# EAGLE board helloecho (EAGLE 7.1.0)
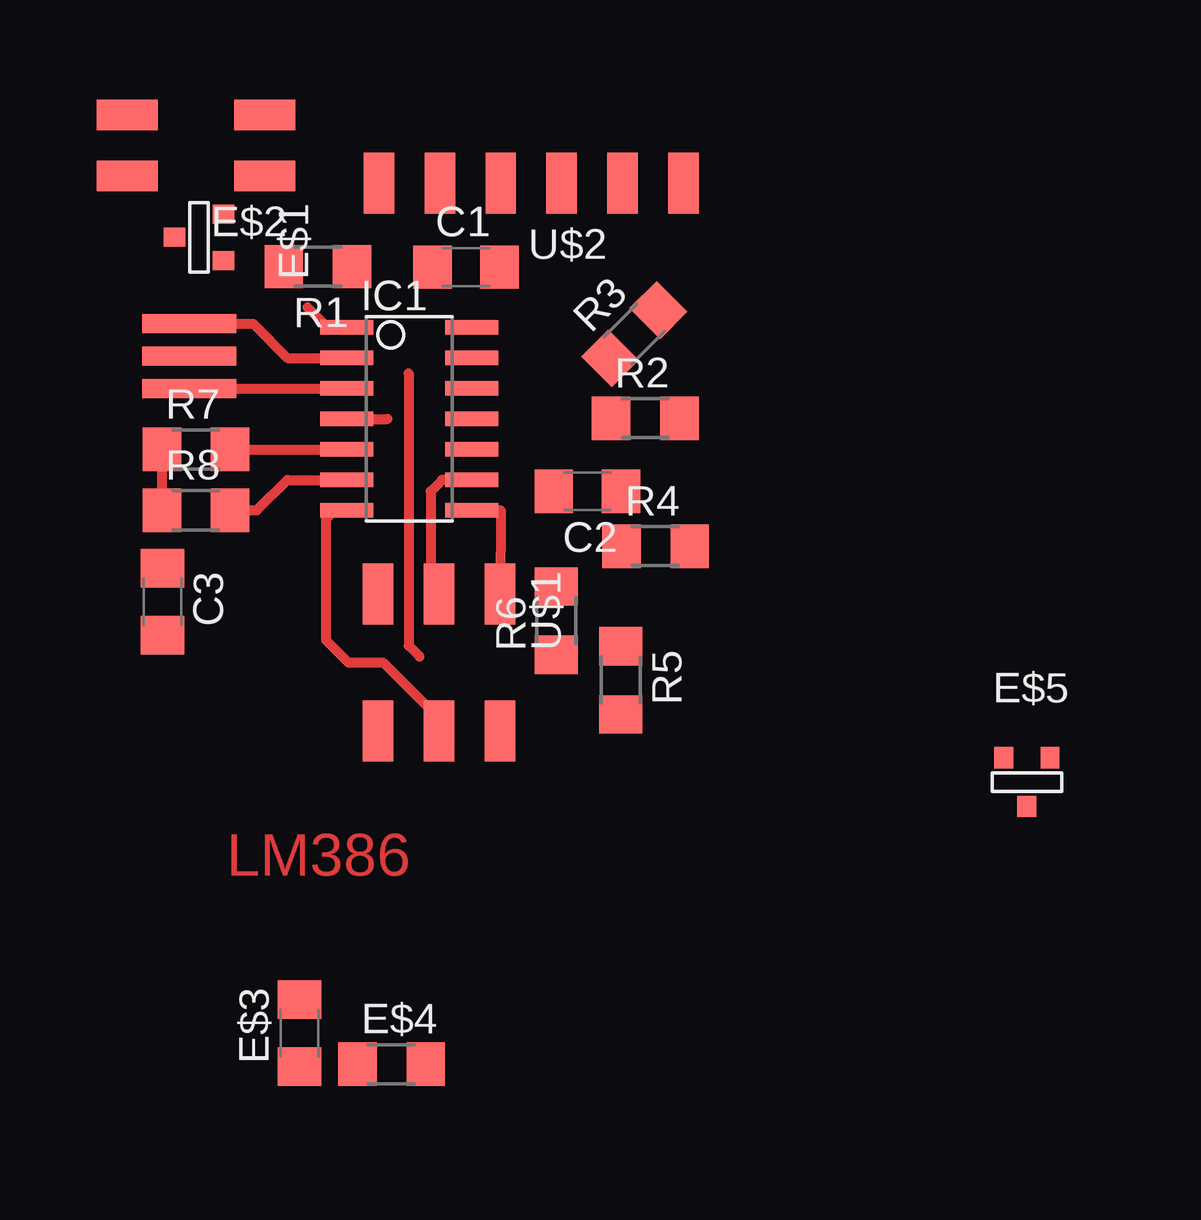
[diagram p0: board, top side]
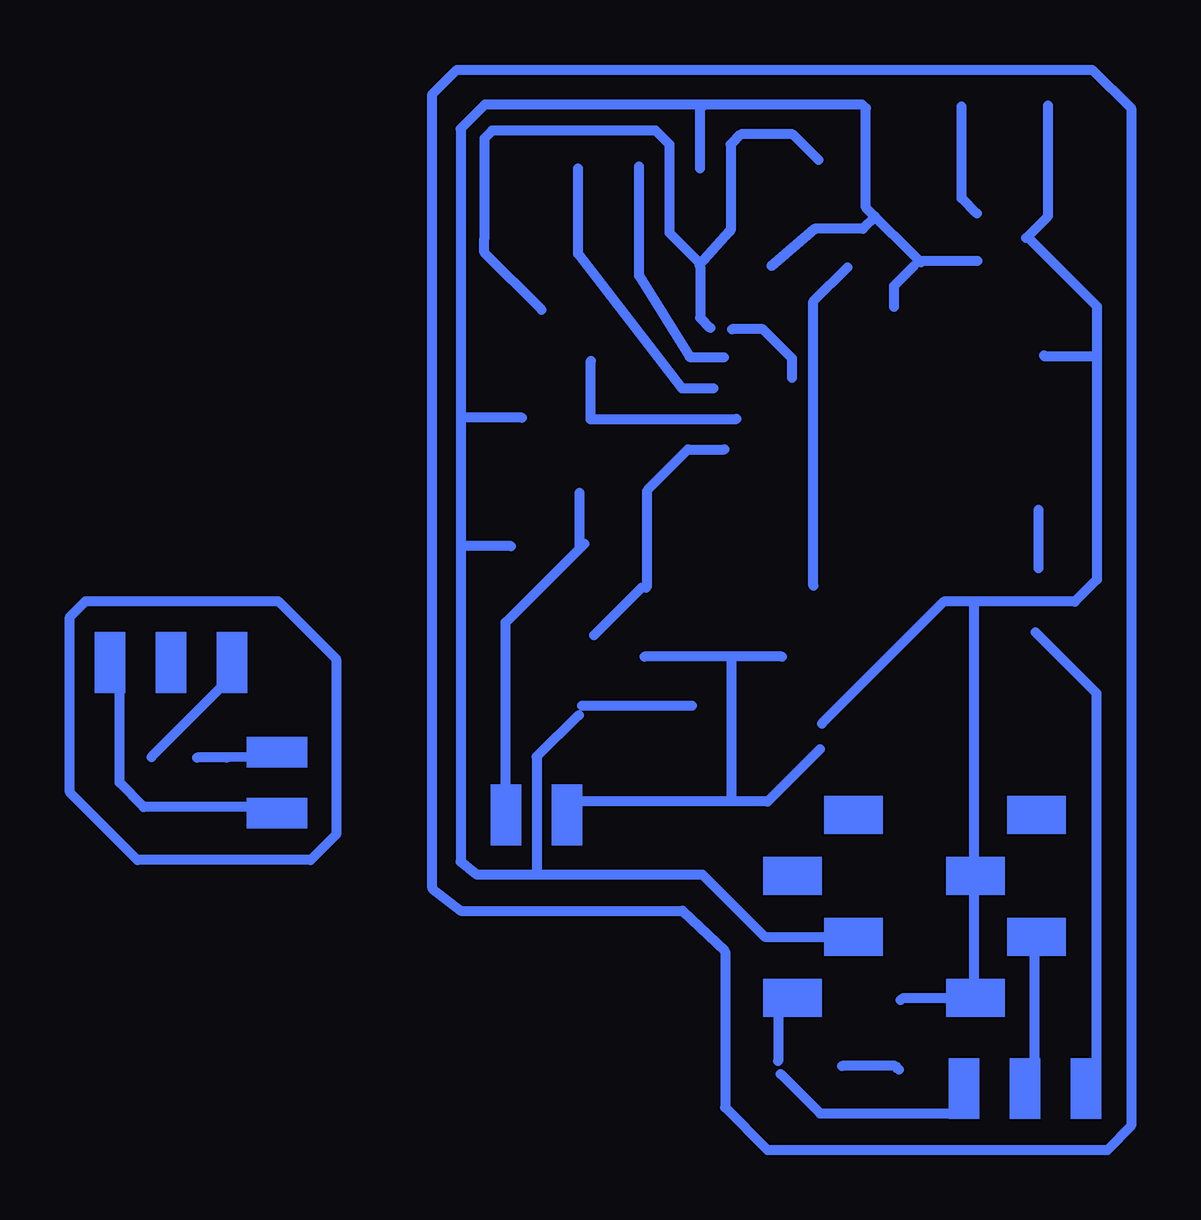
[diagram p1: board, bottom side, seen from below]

No outline drawn. Coordinates in mm, seen from the top.
Copper layers (1*16): Top 0.035mm / dielectric 1.5mm / Bottom 0.035mm
Design rules "default": minimum track width 10mil, minimum drill 24mil, track to track 8mil, track to pad 8mil, pad to pad 8mil, via to via 8mil, smd to smd 8mil, copper to edge 40mil, drill to drill 8mil, minimum pad ring 10mil, minimum via ring 8mil, stop-mask expansion 4mil, vias tented up to drill 0mil, thermal gap 10mil

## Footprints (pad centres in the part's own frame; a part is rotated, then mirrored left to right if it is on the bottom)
EFOBM = smd 0.8 x 3.9: 1 -1.35,0; 2 0,0; 3 1.35,0
C1206 = smd 1.6 x 1.8: 1 -1.4,0; 2 1.4,0
SOT-23 = smd 0.787 x 0.889: 1 0.025,-1.016; 2 -0.94,1.016; 3 0.991,1.016
2X02SMD = smd 2.54 x 1.27: 1 -2.857,1.27; 2 2.857,1.27; 3 -2.857,-1.27; 4 2.857,-1.27
R1206 = smd 1.6 x 1.803: 1 -1.422,0; 2 1.422,0
SOIC14 = smd 0.61 x 2.21: 1 -3.81,-2.603; 2 -2.54,-2.603; 3 -1.27,-2.603; 4 0,-2.603; 5 1.27,-2.603; 6 2.54,-2.603; 7 3.81,-2.603; 8 3.81,2.603; 9 2.54,2.603; 10 1.27,2.603; 11 0,2.603; 12 -1.27,2.603; 13 -2.54,2.603; 14 -3.81,2.603
2X03SMD = smd 2.54 x 1.27: 1 -2.857,2.54; 2 2.857,2.54; 3 -2.857,0; 4 2.857,0; 5 -2.857,-2.54; 6 2.857,-2.54
1X06SMD = smd 2.54 x 1.27: 1 0,6.35; 2 0,3.81; 3 0,1.27; 4 0,-1.27; 5 0,-3.81; 6 0,-6.35

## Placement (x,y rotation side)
20MHZ  RESONATOR  [EFOBM]  18.77,35.64 270 top
C1  1uF  [C1206]  30.3,39.34 0 top
C2  0.1uF  [C1206]  35.36,30 180 top
C3  2.2uF  [C1206]  17.65,25.4 270 top
E$1  REG  [SOT-23]  19.18,40.61 270 top
E$2  [2X02SMD]  19.05,44.42 180 top
E$3  0.1uF  [C1206]  23.37,7.42 90 top
E$4  5  [R1206]  27.2,6.12 0 top
E$5  REG  [SOT-23]  53.64,17.88 0 top
IC1  ATTINY44-SSU  [SOIC14]  27.94,33.02 270 top
R1  10k  [R1206]  24.13,39.37 180 top
R2  10k  [R1206]  37.77,33.05 0 top
R3  10k  [R1206]  37.31,36.55 45 top
R4  10k  [R1206]  38.2,27.71 0 top
R5  10k  [R1206]  36.75,22.12 270 top
R6  10k  [R1206]  34.06,24.61 90 top
R7  1k  [R1206]  19.05,31.75 0 top
R8  255k  [R1206]  19.05,29.21 0 top
U$1  AVRISPSMD  [2X03SMD]  29.18,22.86 270 top
U$2  FTDI-SMD-HEADER  [1X06SMD]  33.02,42.85 90 top

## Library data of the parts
20MHZ C1-C3 E$1-E$5 IC1 R1-R8 U$1 U$2 = fab

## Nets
CTS: U$2.2
MISO: IC1.8 U$1.1
MOSI: IC1.7 U$1.4
N$1: 20MHZ.1 IC1.2
N$2: 20MHZ.3 IC1.3
N$5: R7.1 R8.1
OUT_HI: IC1.5 R7.2
OUT_LO: IC1.6 R8.2
RST: IC1.4
RTS: U$2.6
S$7: IC1.1
S$24: U$1.2
S$36: IC1.14
S$39: U$1.5
SCK: IC1.9 U$1.3

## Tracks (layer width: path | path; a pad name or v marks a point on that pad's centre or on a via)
MISO
  Top 0.406: IC1.8 31.75,29.21 U$1.1
MOSI
  Top 0.406: IC1.7 24.84,29.21 24.46,28.83 24.46,23.8 25.4,22.86 26.85,22.86 29.18,20.52 U$1.4
N$1
  Top 0.406: 20MHZ.1 21.43,36.99 22.86,35.56 IC1.2
N$2
  Top 0.406: 20MHZ.3 IC1.3
N$5
  Top 0.406: R7.1 R8.1
OUT_HI
  Top 0.406: R7.2 IC1.5
OUT_LO
  Top 0.406: R8.2 21.59,29.21 22.86,30.48 IC1.6
RST
  Top 0.406: IC1.4 27.03,33.02
S$1
  Bottom 0.406: 22.55,39.55 24.84,41.83 24.84,45.97 24.99,46.13 40.72,46.13 41.73,45.11 41.73,14.55 41.05,14.02 31.65,14.02 29.06,11.43 25.3,11.43
S$2
  Bottom 0.406: 37.19,17.12 37.31,17.25
S$3
  Bottom 0.406: 18.11,40.62 15.21,37.72 15.21,26.31 16.13,25.4 20.32,25.4 | 20.32,25.4 21.59,25.4 26.67,20.32 | 20.32,9.53 20.32,25.4
S$4
  Bottom 0.406: 39.62,27.71 41.68,27.71
S$5
  Bottom 0.406: 26.75,19.25 28.93,17.07 37.26,17.07 37.31,17.02
S$6
  Bottom 0.406: 17.78,24.13 15.24,21.59 15.24,5.08
S$7
  Top 0.406: IC1.1 24.54,36.83 23.7,37.67
S$8
  Bottom 0.406: 28.78,39.4 26.98,40.95 24.97,40.95 24.46,41.45
S$9
  Bottom 0.406: 25.6,39.34 27.03,37.92 27.03,26.06
S$10
  Top 0.406: 27.91,34.92 27.91,23.57 28.37,23.11
S$11
  Bottom 0.406: 39.85,16.51 39.85,24.54 36.58,27.81
S$12
  Bottom 0.406: 33.91,30.1 32.26,31.75 30.73,31.75
S$13
  Bottom 0.406: 22.86,39.37 23.67,38.56 23.67,37.69
S$14
  Bottom 0.406: 18.16,40.56 17.25,41.48 17.25,46.08
S$15
  Bottom 0.406: 20.52,8.87 23.32,8.87 23.39,8.79
S$16
  Bottom 0.406: 32.16,35.59 30.76,35.59
S$17
  Bottom 0.406: 31.19,34.29 32.49,34.29 | 32.49,34.29 32.51,34.29 | 32.49,34.29 36.83,39.9 36.83,43.46
S$18
  Bottom 0.406: 36.3,35.43 36.32,35.41 36.32,32.99
S$19
  Bottom 0.406: 28.35,23.11 34.06,23.11
S$20
  Bottom 0.406: 32.08,21.06 36.68,21.06
S$21
  Bottom 0.406: 39.88,16.61 39.85,16.64
S$22
  Bottom 0.406: 31.75,39.37 31.75,37.24 31.32,36.8
S$23
  Bottom 0.406: 20.19,39.6 22.68,39.6
S$24
  Top 0.406: U$1.2 31.73,19.43
S$25
  Bottom 0.406: 30.5,23.06 30.45,23.01 30.45,17.2
S$26
  Bottom 0.406: 36.17,24 34.19,25.98
S$27
  Bottom 0.406: 31.77,39.52 33.02,40.77 33.02,44.45 33.6,45.03 40.41,45.03 40.74,44.7 40.74,41.66 40.74,40.56 40.74,39.95 38.35,37.57
S$28
  Bottom 0.406: 30.5,40.84 31.77,39.42
S$29
  Bottom 0.406: 32.18,35.61 34.29,38.99 34.29,43.54
S$30
  Bottom 0.406: 23.47,5.89 23.62,6.04 25.83,6.04
S$31
  Bottom 0.406: 17.42,35.66 17.4,35.64 15.32,35.64
S$32
  Bottom 0.406: 36.78,29.95 36.78,27.64
S$33
  Bottom 0.406: 14.78,2.54 13.79,3.56 13.79,45.97 15.42,47.57 41.88,47.57 42.9,46.56 42.9,13.46
S$34
  Bottom 0.406: 17.8,5.21 17.8,11.51
S$35
  Bottom 0.406: 20.22,41.58 20.85,42.22 20.85,46.05
S$36
  Top 0.406: IC1.14 31.42,36.83
S$37
  Bottom 0.406: 27.91,34.72 27.91,35.53 29.13,36.75 30.43,36.75
S$38
  Bottom 0.406: 34.01,25.98 33.96,26.04 33.96,30
S$39
  Top 0.406: 27.05,26.23 U$1.5
S$40
  Bottom 0.406: 31.75,43.46 31.75,45.95 31.67,46.02
S$41
  Bottom 0.406: 17.65,29.23 17.65,26.8
S$42
  Bottom 0.406: 28.68,8.71 28.5,8.53 28.5,6.25
S$43
  Bottom 0.406: 28.4,5.71 26.75,4.06 20.65,4.06
S$44
  Bottom 0.406: 36.8,20.68 38.56,18.95 38.56,14.1
S$45
  Bottom 0.406: 51.16,22.55 51.16,22.38 54.61,18.92
S$46
  Bottom 0.406: 26.82,43.81 27.89,44.88 30.05,44.88 30.48,44.45 30.48,40.87
S$47
  Bottom 0.406: 36.3,32.99 36.27,33.02 30.23,33.02
S$48
  Bottom 0.406: 39.17,33.07 41.6,33.07
S$49
  Bottom 0.406: 42.9,13.44 41.73,12.52 32.49,12.52 30.71,10.82 30.71,4.32 28.93,2.54 14.81,2.54
S$50
  Bottom 0.406: 49,16.38 49.81,16.84 54.94,16.84 55.93,17.86 55.93,21.67
S$51
  Bottom 0.406: 48.9,18.95 51.49,18.9 52.7,18.9
S$53
  Bottom 0.406: 46.91,22.99 46.91,15.7 47.98,14.63 55.19,14.63 58.01,17.45 58.01,24.77 57.35,25.43 49.33,25.43 46.91,23.01
SCK
  Top 0.406: IC1.9 29.31,30.48 28.83,30 28.83,25.95 U$1.3
(copper drawn outside any net)
  shapes: Bottom area x18

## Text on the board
Top: LM386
